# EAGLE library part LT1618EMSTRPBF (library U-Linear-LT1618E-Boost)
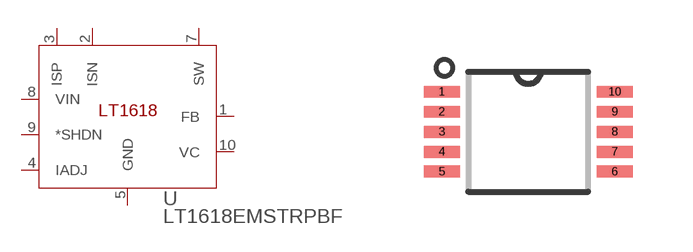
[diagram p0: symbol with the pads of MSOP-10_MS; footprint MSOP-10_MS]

Designator prefix U

## LT1618EMSTRPBF (DESCRIPTION: PMIC - DC/DC voltage regulator Linear Technology LT1618EMS#TRPBF Converter, Boost, Converter/amplifier, SEPIC MSOP 10; DIGI-KEY_PART_NUMBER: LT1618EMS#TRPBFCT-ND; DIGI-KEY_PURCHASE_URL: https://www.digikey.com/product-detail/en/linear-technology-analog-devices/LT1618EMS-TRPBF/LT1618EMS-TRPBFCT-ND/3885220?utm_source=snapeda&utm_medium=aggregator&utm_campaign=symbol; MF: Linear Technology/Analog; MP: LT1618EMS#TRPBF; PACKAGE: MSOP-10 Linear Technology)  [MSOP-10_MS]
1  FB  in
2  ISN  pas
3  ISP  pas
4  IADJ  in
5  GND  pwr
7  SW  out
8  VIN  pwr
9  *SHDN  in
10  VC  pas

## Footprint MSOP-10_MS (pad centres in mm)
smd 0.9 x 0.3: 1 -2.165,1; 2 -2.165,0.5; 3 -2.165,0; 4 -2.165,-0.5; 5 -2.165,-1; 6 2.165,-1; 7 2.165,-0.5; 8 2.165,0; 9 2.165,0.5; 10 2.165,1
